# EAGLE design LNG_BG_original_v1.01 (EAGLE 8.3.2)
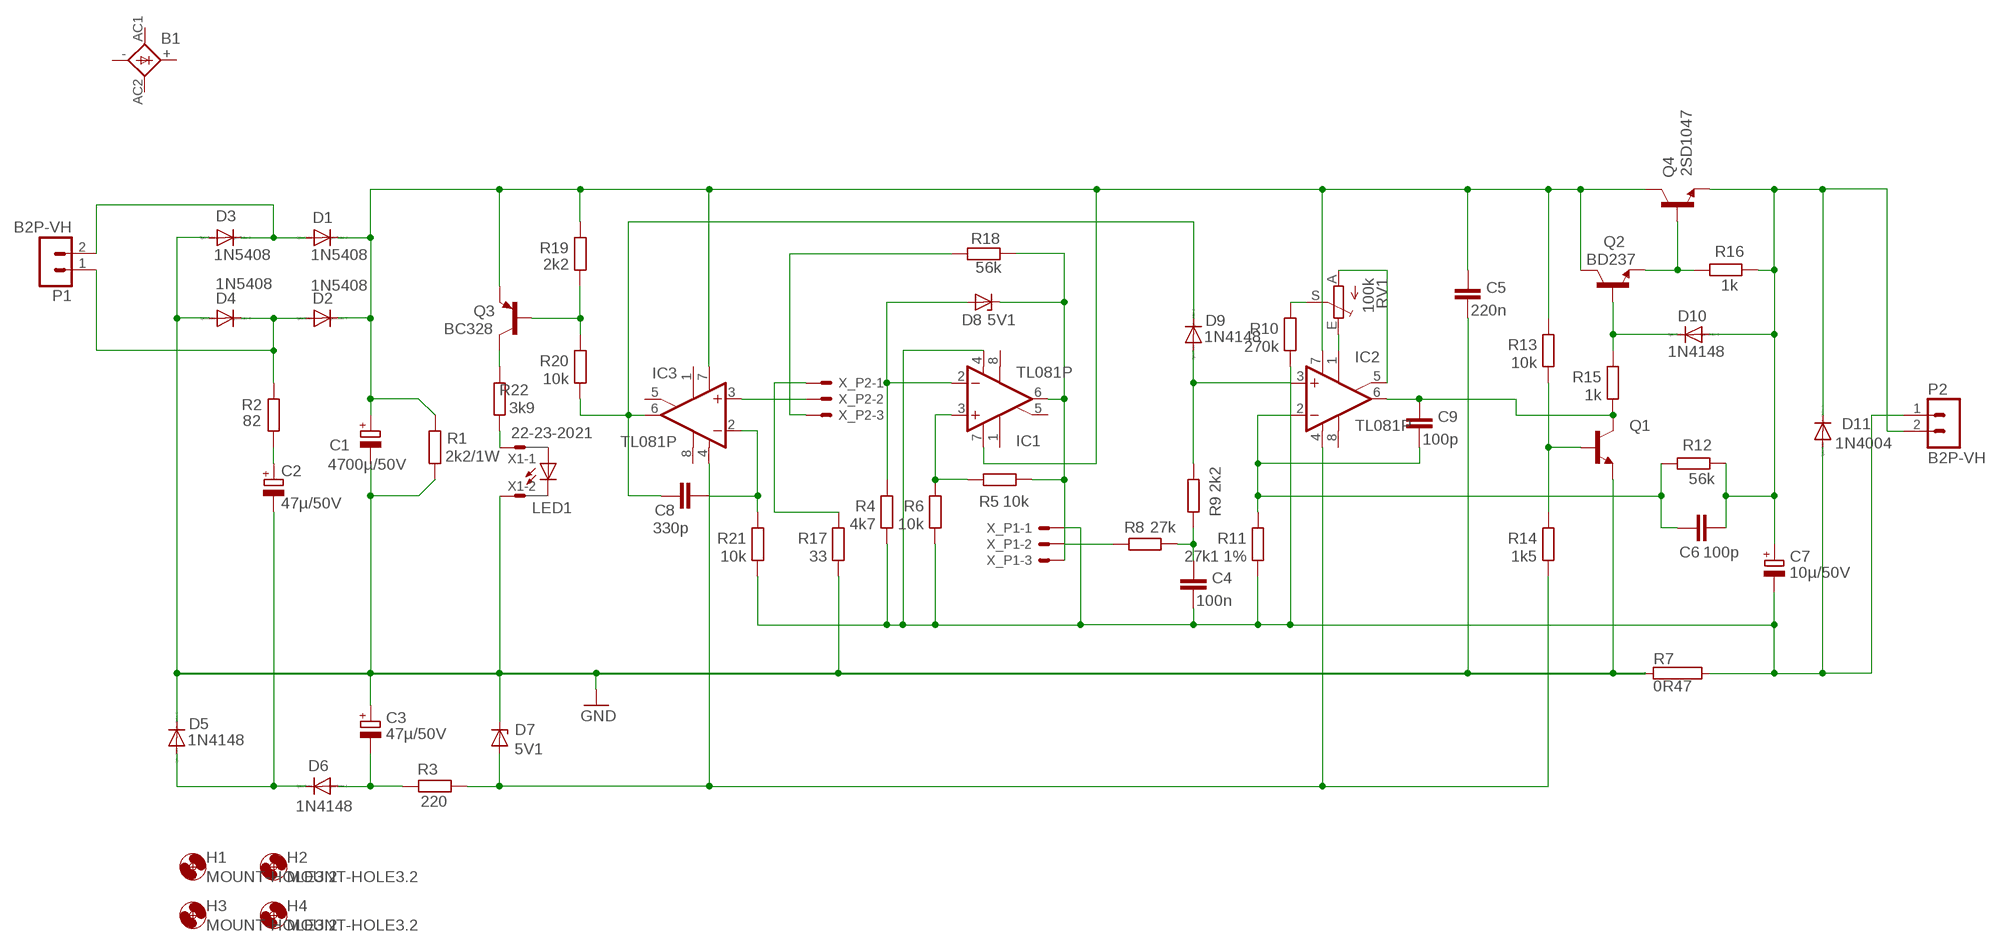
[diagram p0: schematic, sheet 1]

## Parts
B1  DSI32A  [DSI32A]
C1  4700µ/50V  CPOL-EUE7.5-18  [E7,5-18]
C2  47µ/50V  CPOL-EUE2.5-6  [E2,5-6]
C3  47µ/50V  CPOL-EUE2.5-6  [E2,5-6]
C4  100n  C-EU050-024X044  [C050-024X044]
C5  220n  C-EU050-024X044  [C050-024X044]
C6  100p  C-EU050-024X044  [C050-024X044]
C7  10µ/50V  CPOL-EUE2.5-6  [E2,5-6]
C8  330p  C-EU050-024X044  [C050-024X044]
C9  100p  C-EU050-024X044  [C050-024X044]
D1  1N5408  1N5400  [DO201-15]
D2  1N5408  1N5400  [DO201-15]
D3  1N5408  1N5400  [DO201-15]
D4  1N5408  1N5400  [DO201-15]
D5  1N4148  1N4148DO35-10  [DO35-10]
D6  1N4148  1N4148DO35-10  [DO35-10]
D7  5V1  BZV10  [DO34Z7]
D8  5V1  BZV10  [DO34Z7]
D9  1N4148  1N4148DO35-10  [DO35-10]
D10  1N4148  1N4148DO35-10  [DO35-10]
D11  1N4004  [DO41-10]
H1  MOUNT-HOLE3.2  [3,2]
H2  MOUNT-HOLE3.2  [3,2]
H3  MOUNT-HOLE3.2  [3,2]
H4  MOUNT-HOLE3.2  [3,2]
IC1  TL081P  [DIL08]
IC2  TL081P  [DIL08]
IC3  TL081P  [DIL08]
LED1  LED3MM  [LED3MM]
P1  B2P-VH  [B2P-VH]
P2  B2P-VH  [B2P-VH]
Q1  BC337-NPN-TO92-CBE  [TO92-CBE]
Q2  BD237  BD235  [TO126]
Q3  BC328  [TO92-EBC]
Q4  2SD1047  2SC3855  [SC-65]
R1  2k2/1W  R-EU_0414/15  [0414/15]
R2  82  R-EU_0207/10  [0207/10]
R3  220  R-EU_0207/10  [0207/10]
R4  4k7  R-EU_0207/10  [0207/10]
R5  10k  R-EU_0207/10  [0207/10]
R6  10k  R-EU_0207/10  [0207/10]
R7  0R47  RKH208-8  [KH208-8]
R8  27k  R-EU_0207/10  [0207/10]
R9  2k2  R-EU_0207/10  [0207/10]
R10  270k  R-EU_0207/10  [0207/10]
R11  27k1 1%  R-EU_0207/10  [0207/10]
R12  56k  R-EU_0207/10  [0207/10]
R13  10k  R-EU_0207/10  [0207/10]
R14  1k5  R-EU_0207/10  [0207/10]
R15  1k  R-EU_0207/10  [0207/10]
R16  1k  R-EU_0207/10  [0207/10]
R17  33  R-EU_0207/10  [0207/10]
R18  56k  R-EU_0207/10  [0207/10]
R19  2k2  R-EU_0207/10  [0207/10]
R20  10k  R-EU_0207/10  [0207/10]
R21  10k  R-EU_0207/10  [0207/10]
R22  3k9  R-EU_0207/10  [0207/10]
RV1  100k  TRIM_EU-B64Y  [B64Y]
X1  22-23-2021  [22-23-2021]
X_P1  22-23-2031  [22-23-2031]
X_P2  22-23-2031  [22-23-2031]

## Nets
GND: C1.- C3.+ C5.2 D3.A D4.A D5.C D7.C Q1.E R1.1 R7.1 R17.1 X1.2
N$1: D1.A D3.C P1.2
N$2: D2.A D4.C P1.1 R2.1
N$3: C2.+ R2.2
N$4: C9.1 IC2.6(OUT) Q1.C R15.1
N$5: C2.- D5.A D6.C
N$6: Q3.B R19.1 R20.2
N$7: C3.- D6.A R3.1
N$8: C1.+ C5.1 D1.C D2.C IC1.7(V+) IC2.7(V+) IC3.7(V+) Q2.2(C) Q3.E Q4.2(C) R1.2 R13.2 R19.2
N$9: C8.2 D9.C IC3.6(OUT) R20.1
N$10: C8.1 IC3.2(-IN) R21.2
N$11: R22.1 X1.1
N$12: Q3.C R22.2
N$13: D7.A IC2.4(V-) IC3.4(V-) R3.2 R14.1
N$14: IC3.3(+IN) X_P2.2
N$15: R17.2 X_P2.1
N$16: R18.2 X_P2.3
N$17: IC1.3(+IN) R5.2 R6.2
N$18: R8.2 X_P1.2
N$19: D8.A IC1.2(-IN) R4.2
N$20: D8.C IC1.6(OUT) R5.1 R18.1 X_P1.3
N$21: C4.1 R8.1 R9.2
N$22: D9.A IC2.3(+IN) R9.1
N$23: C6.2 C7.+ D10.A D11.C P2.2 Q4.3(E) R12.1 R16.1
N$24: R10.2 RV1.S
N$25: IC2.1(ON1) RV1.E
N$26: IC2.5(ON2) RV1.A
N$28: Q1.B R13.1 R14.2
N$29: D10.C Q2.3(B) R15.2
N$31: Q2.1(E) Q4.1(B) R16.2
N$32: C4.2 C7.- D11.A IC1.4(V-) P2.1 R4.1 R6.1 R7.2 R10.1 R11.1 R21.1 X_P1.1
N$35: C6.1 C9.2 IC2.2(-IN) R11.2 R12.2
Unconnected: B1.+ B1.- B1.AC1 B1.AC2 IC1.1(ON1) IC1.5(ON2) IC1.8(OPT) IC2.8(OPT) IC3.1(ON1) IC3.5(ON2) IC3.8(OPT) LED1.A LED1.K(C)

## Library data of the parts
B1 = rectifier:DSI32A: RECTIFIER 3.2 A
C1-C3 C7 = rcl:CPOL-EU: POLARIZED CAPACITOR, European symbol
C4-C6 C8 C9 = rcl:C-EU: CAPACITOR, European symbol
D1-D4 = diode:1N5400: DIODE
D5 D6 D9 D10 = diode:1N4148: DIODE
D7 D8 = diode:BZV10: Z DIODE
D11 = diode:1N4004: DIODE
H1-H4 = holes:MOUNT-HOLE: MOUNTING HOLE with drill center marker
IC1-IC3 = linear:TL081: OP AMP
LED1 = led:LED: LED
P1 P2 = con-jst-vh:B2P-VH: HEADER
Q1 = transistor:*-NPN-: NPN Transistror BF959 corrected 2008.03.06
Q2 = transistor:BD235: NPN TRANSISTOR
Q3 = transistor-pnp:BC328*: PNP Transistror
Q4 = transistor-JP:2SC3855: NPN Power Transistor 140V, 10A, 100W
R1-R6 R8-R22 = rcl:R-EU_: RESISTOR, European symbol
R7 = resistor-power:R: Power Resitor; OC_FARNELL: unknown; OC_NEWARK: unknown
RV1 = pot:TRIM_EU-: POTENTIOMETER
X1 = con-molex:22-23-2021: .100" (2.54mm) Center Header - 2 Pin; MF: MOLEX; MPN: 22-23-2021; OC_FARNELL: 1462926; OC_NEWARK: 25C3832
X_P1 X_P2 = con-molex:22-23-2031: .100" (2.54mm) Center Header - 3 Pin; MF: MOLEX; MPN: 22-23-2031; OC_FARNELL: 1462950; OC_NEWARK: 30C0862

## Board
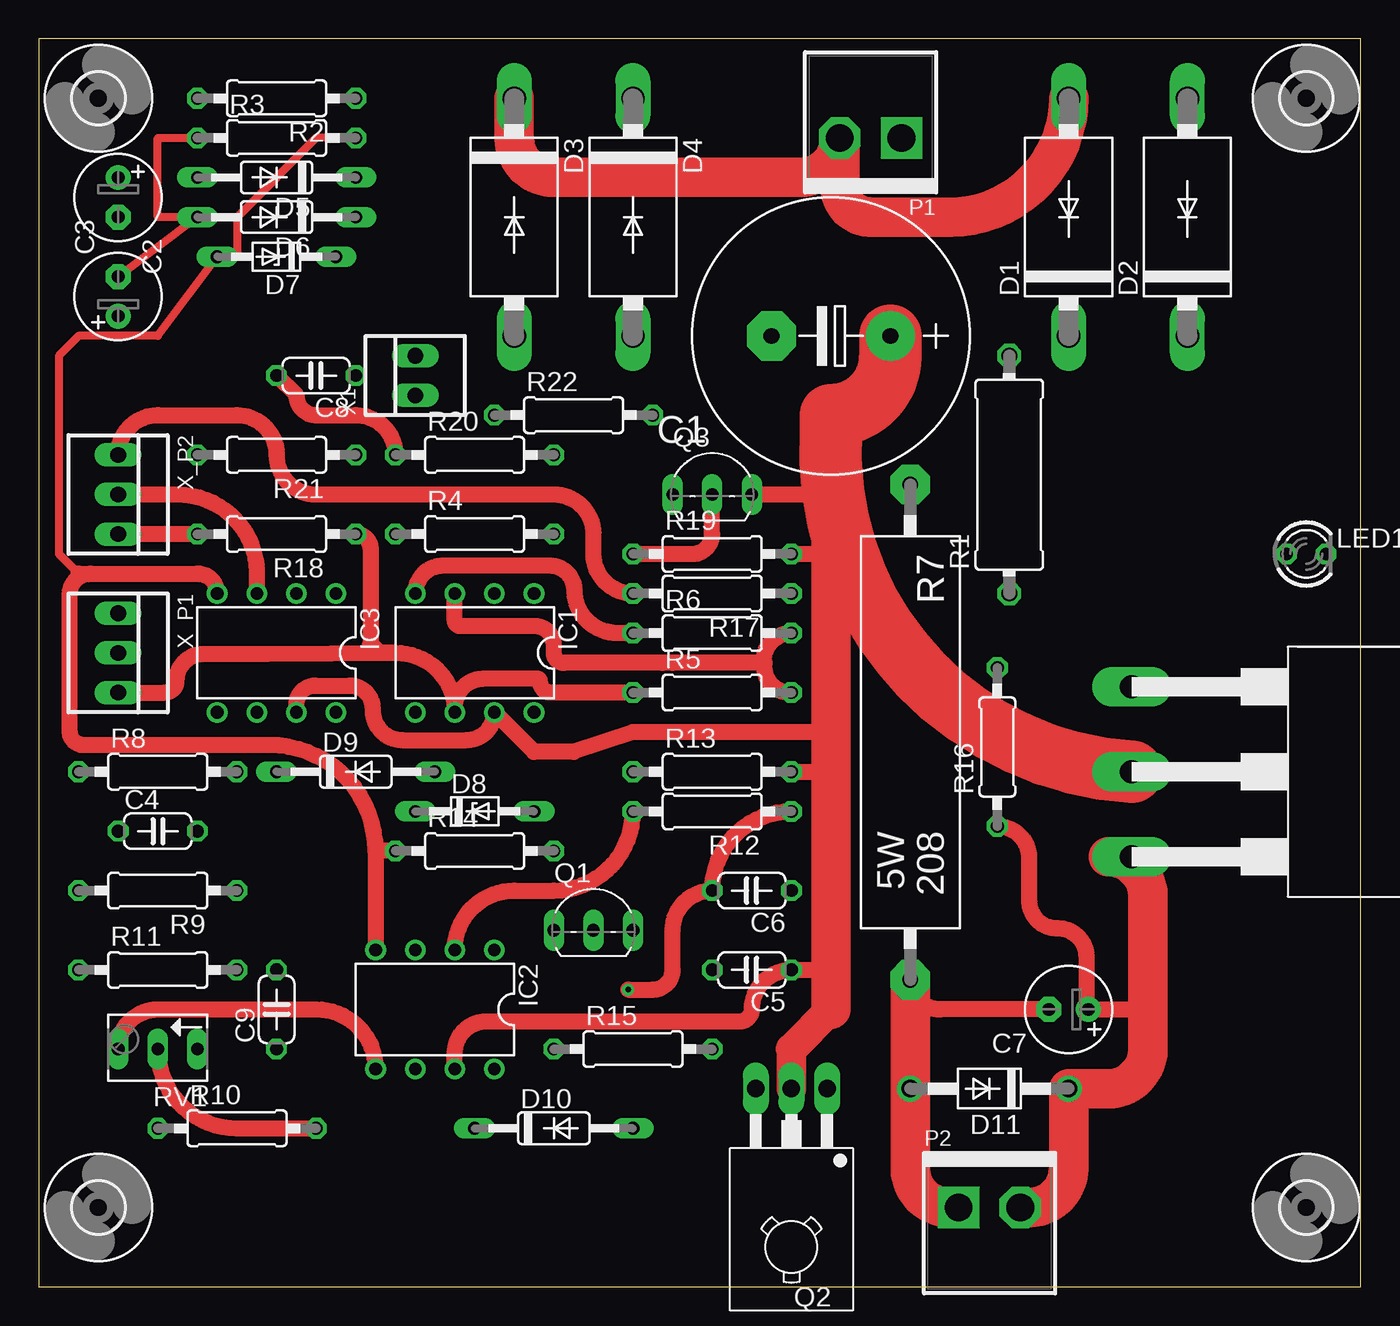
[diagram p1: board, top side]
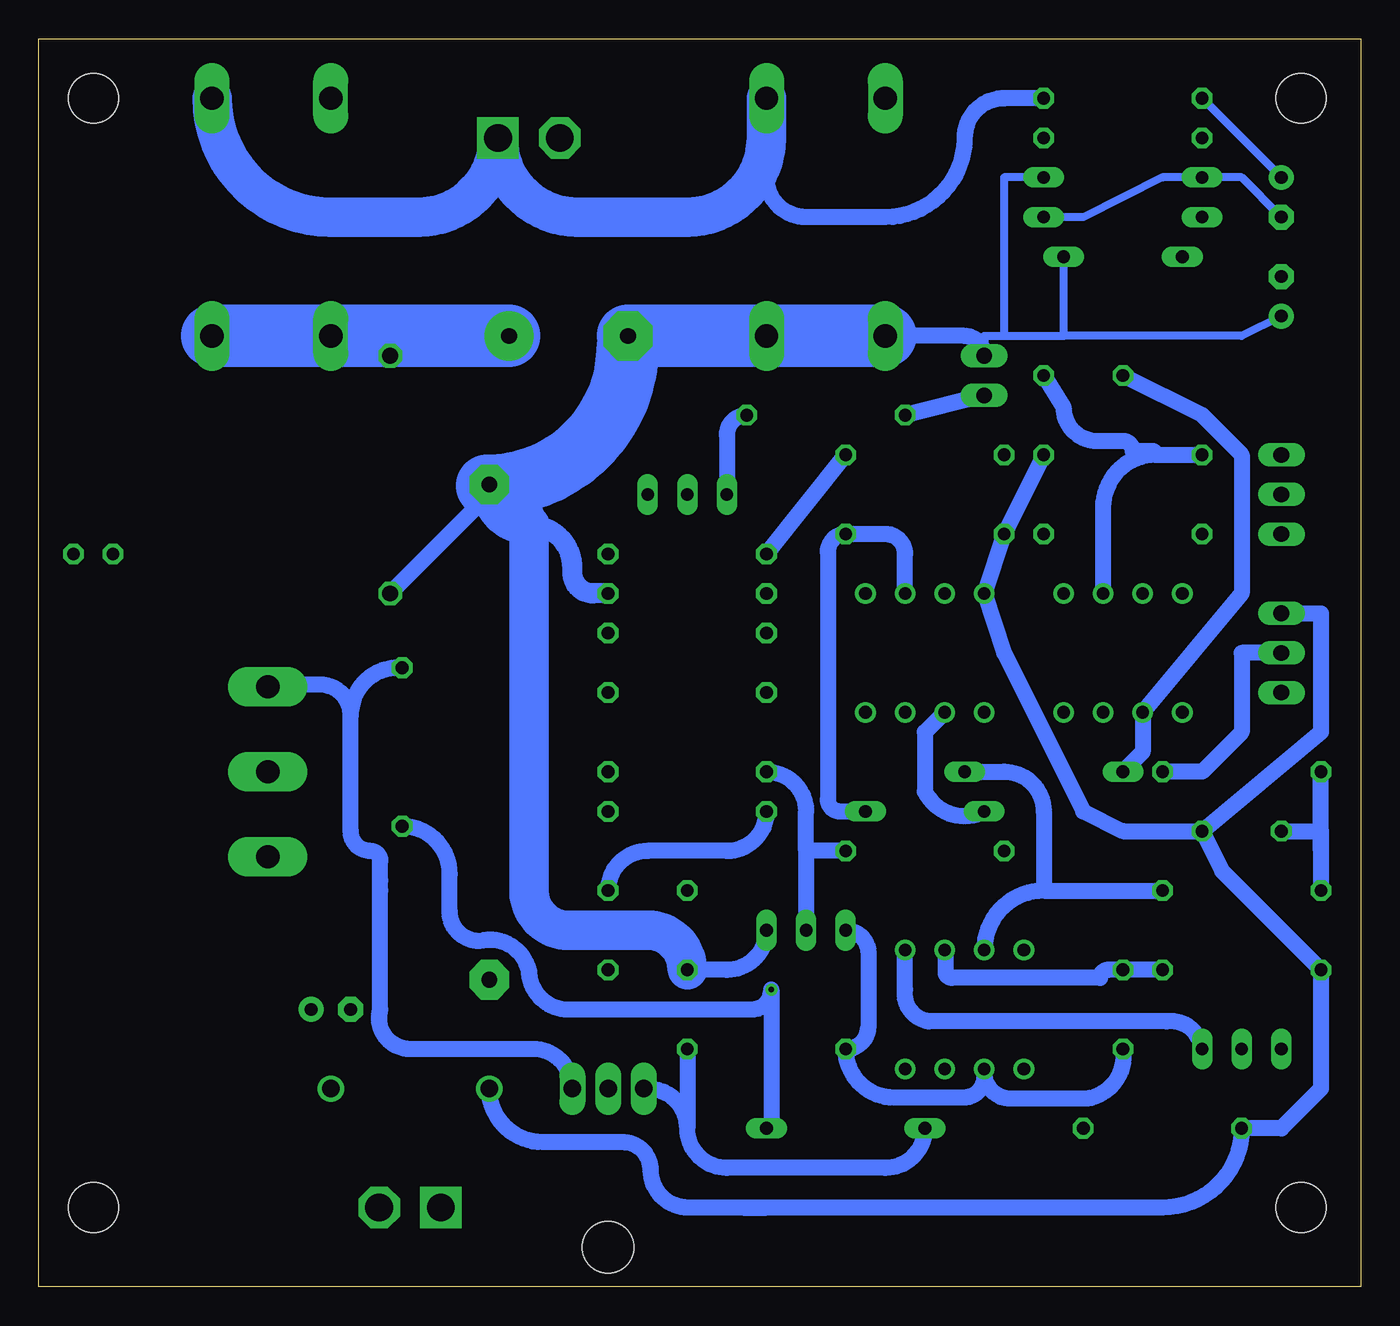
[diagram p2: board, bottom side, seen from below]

Size 84.76 x 80 mm. Coordinates in mm from the lower left corner, seen from the top.
Outline: 0,0 84.76,0 84.76,80 0,80 0,0
Copper layers (1*16): Top 0.035mm / dielectric 1.5mm / Bottom 0.035mm
Design rules "default": minimum track width 6mil, minimum drill 0.35mm, track to track 6mil, track to pad 6mil, pad to pad 6mil, via to via 6mil, smd to smd 6mil, copper to edge 40mil, drill to drill 6mil, minimum pad ring 10mil, minimum via ring 8mil, stop-mask expansion 4mil, vias tented up to drill 0mil, thermal gap 10mil

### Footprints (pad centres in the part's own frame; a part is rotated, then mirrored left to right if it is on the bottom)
DSI32A = drill 1.321 long: + -3.982,1.5; - 11.004,1.5; AC1 -11.5,1.5; AC2 3.511,1.5
E7,5-18 = drill 1.016 pad 3.15: + -3.81,0 | drill 1.016 pad 3.15 octagon: - 3.81,0
E2,5-6 = drill 0.813 pad 1.6: + -1.27,0 | drill 0.813 pad 1.6 octagon: - 1.27,0
C050-024X044 = drill 0.813 octagon: 1 -2.54,0; 2 2.54,0
DO201-15 = drill 1.499 long: A 7.62,0; C -7.62,0
DO35-10 = drill 0.813 long: A 5.08,0; C -5.08,0
DO34Z7 = drill 0.813 long: A 3.81,0; C -3.81,0
DO41-10 = drill 1.118: A 5.08,0; C -5.08,0
3,2 = hole 3.2: 0,0
DIL08 = drill 0.813 pad 1.27: 1 -3.81,-3.81; 2 -1.27,-3.81; 3 1.27,-3.81; 4 3.81,-3.81; 5 3.81,3.81; 6 1.27,3.81; 7 -1.27,3.81; 8 -3.81,3.81
LED3MM = drill 0.813 octagon: A -1.27,0; K 1.27,0
B2P-VH = drill 1.778 square: 1 -1.98,0 | drill 1.778 octagon: 2 1.98,0
TO92-CBE = drill 0.813 long: B 0,0; C -2.54,0; E 2.54,0
TO126 = drill 1.118 long: 1 -2.286,-5.08; 2 0,-5.08; 3 2.286,-5.08 | hole 3.302: 0,5.08
TO92-EBC = drill 0.813 long: B 0,-1.27; C -2.54,-1.27; E 2.54,-1.27
SC-65 = drill 1.5 pad 2.54 long: 1 -5.45,-18.81; 2 0,-18.81; 3 5.45,-18.81
0414/15 = drill 1.016 octagon: 1 -7.62,0; 2 7.62,0
0207/10 = drill 0.813 octagon: 1 -5.08,0; 2 5.08,0
KH208-8 = drill 1.016 pad 2.54 octagon: 1 -15.875,0; 2 15.875,0
B64Y = drill 0.813 long: A 2.54,0; E -2.54,0; S 0,0
22-23-2021 = drill 1 long: 1 -1.27,0; 2 1.27,0
22-23-2031 = drill 1 long: 1 -2.54,0; 2 0,0; 3 2.54,0

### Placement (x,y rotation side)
B1  not placed on the board
C1  50.8,60.96 180 top
C2  5.08,69.85 270 top
C3  5.08,63.5 90 top
C4  7.62,29.21 0 top
C5  45.72,20.32 180 top
C6  45.72,25.4 180 top
C7  66.04,17.78 180 top
C8  17.78,58.42 180 top
C9  15.24,17.78 90 top
D1  66.04,68.58 90 top
D2  73.66,68.58 90 top
D3  30.48,68.58 270 top
D4  38.1,68.58 270 top
D5  15.24,71.12 180 top
D6  15.24,68.58 180 top
D7  15.24,66.04 180 top
D8  27.94,30.48 0 top
D9  20.32,33.02 0 top
D10  33.02,10.16 0 top
D11  60.96,12.7 180 top
H1  3.81,76.2 0 top
H2  3.81,5.08 0 top
H3  81.28,5.08 0 top
H4  81.28,76.2 0 top
IC1  27.94,40.64 180 top
IC2  25.4,17.78 180 top
IC3  15.24,40.64 180 top
LED1  81.28,46.99 0 top
P1  53.34,73.66 180 top
P2  60.96,5.08 0 top
Q1  35.56,22.86 0 top
Q2  48.26,7.62 180 top
Q3  43.18,52.07 0 top
Q4  88.9,33.02 270 top
R1  62.23,52.07 90 top
R2  15.24,76.2 180 top
R3  15.24,73.66 0 top
R4  27.94,48.26 0 top
R5  43.18,38.1 0 top
R6  43.18,41.91 0 top
R7  55.88,35.56 270 top
R8  7.62,33.02 0 top
R9  7.62,25.4 180 top
R10  12.7,10.16 0 top
R11  7.62,20.32 0 top
R12  43.18,30.48 180 top
R13  43.18,33.02 0 top
R14  27.94,27.94 0 top
R15  38.1,15.24 0 top
R16  61.47,34.61 90 top
R17  43.18,44.45 180 top
R18  15.24,48.26 180 top
R19  43.18,46.99 0 top
R20  27.94,53.34 0 top
R21  15.24,53.34 180 top
R22  34.29,55.88 0 top
RV1  7.62,15.24 180 top
X1  24.13,58.42 90 top
X_P1  5.08,40.64 270 top
X_P2  5.08,50.8 270 top

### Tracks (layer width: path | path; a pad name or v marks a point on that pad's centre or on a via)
GND
  Bottom 0.508: C3.+ 7.62,60.96 19.05,60.96 | 22.86,60.96 19.05,60.96 | 22.86,60.96 24.13,60.96 X1.2 | D7.C 19.05,60.96 | D5.C 22.86,71.12 22.86,60.96
  Bottom 1.016: R1.1 55.88,50.8 R7.1 arc-90 55.37,50.93 | Q1.E arc90 40.64,20.32 C5.2 | X1.2 arc-90 25.4,60.96 D3.A
  Bottom 1.27: R17.1 49.21,44.45 arc90 50.55,45.78 50.55,46.1 arc-90 53.28,48.83
  Bottom 2.54: C1.- 46.99,60.33 | 56.01,51.37 R7.1 arc-90 53.28,48.83 | C5.2 arc-90 45.72,22.86 50.8,22.86 arc90 53.34,25.4 53.34,48.26 arc-90 55.88,50.8
  Bottom 4: D3.A D4.A C1.- | 56.01,51.37 arc-90 46.99,60.33
N$1
  Top 2.54: D3.C 30.48,73.66 arc90 33.02,71.12 48.82,71.12 arc90 P1.2 51.36,70.56 arc90 53.34,68.58 58.42,68.58 arc90 D1.A
N$2
  Bottom 1.016: R2.1 22.86,76.2 arc-90 25.4,73.66 arc90 30.48,68.58 35.56,68.58 arc90 38.1,71.12 38.1,73.66
  Bottom 2.54: D2.A arc-90 66.04,68.58 60.4,68.58 arc-90 P1.1 arc-90 50.24,68.58 43.18,68.58 arc-90 38.1,73.66 D4.C
N$3
  Bottom 0.508: R2.2 C2.+
N$4
  Bottom 1.016: C9.1 arc90 17.53,12.06 22.61,12.06 arc90 IC2.6 24.13,13.46 arc90 25.46,12.13 29.91,12.13 arc90 R15.1 arc-90 31.56,16.7 31.56,21.4 arc-90 Q1.C
N$5
  Bottom 0.508: C2.- 7.62,71.12 D5.A 12.7,71.12 17.78,68.58 D6.C
N$6
  Top 1.016: R19.1 41.91,46.99 arc90 43.18,48.26 Q3.B
  Bottom 1.016: R20.2 R19.1
N$7
  Top 0.508: C3.- D6.A 7.62,68.58 7.62,73.66 R3.1
N$8
  Top 1.016: R19.2 50.8,46.99 | R13.2 50.8,33.02 | 50.8,35.56 38.1,35.56 34.29,34.29 31.75,34.29 IC1.7 arc-90 27.43,35.05 23.3,35.05 arc-90 21.4,36.96 21.4,37.08 arc90 19.94,38.54 17.72,38.54 arc90 16.51,37.34 IC3.7 | IC2.7 26.67,14.99 arc-90 28.7,17.02 44.96,17.02 arc90 45.72,17.78 arc-90 C5.1 50.8,20.32 | Q3.E 50.8,50.8
  Top 1.9: Q2.2 48.26,15.24
  Top 2: 50.8,17.78 48.26,15.24
  Top 2.54: 50.8,54.85 50.8,50.8 50.8,46.99 50.8,35.56 50.8,33.02 50.8,20.32 50.8,17.78
  Top 4: Q4.2 arc-90 50.8,54.85 50.8,55.88 arc90 54.61,59.69 C1.+
  Bottom 1.016: R1.2 arc-90 63.5,60.96
  Bottom 4: D2.C D1.C 63.5,60.96 C1.+
N$9
  Top 1.016: C8.2 16.51,57.15 arc90 17.78,55.88 20.32,55.88 arc-90 R20.1
  Bottom 1.016: D9.C 13.97,34.29 IC3.6 7.62,44.45 7.62,53.34 10.16,55.88 C8.2
N$10
  Bottom 1.016: 13.14,53.34 R21.2 | 13.14,53.34 arc-90 16.51,49.97 IC3.2 | C8.1 19.05,56.39 arc-90 16.89,54.23 15.24,54.23 arc90 14.61,53.59 13.4,53.59 arc90 13.14,53.34
N$11
  Bottom 1.016: X1.1 R22.1
N$12
  Bottom 1.016: R22.2 arc-90 40.64,54.61 Q3.C
N$13
  Top 0.508: R3.2 17.78,73.66 12.7,68.58 12.7,66.04 D7.A 7.62,60.96 2.54,60.96 1.27,59.69 1.27,46.99 2.54,45.72 3.3,45.72
  Top 1.016: 21.59,27.94 IC2.4 | 21.59,27.94 arc90 14.8,34.73 2.86,34.73 arc-90 1.97,35.62 1.97,44.39 arc-90 3.3,45.72 | 2.54,45.72 10.16,45.72 arc-90 IC3.4 | R14.1 21.59,27.94
N$14
  Top 1.016: X_P2.2 8.89,50.8 arc-90 13.97,45.72 IC3.3
N$15
  Top 1.016: R17.2 arc-90 35.56,46.99 35.56,48.26 arc90 33.02,50.8 17.78,50.8 arc-90 15.24,53.34 arc90 12.7,55.88 7.62,55.88 arc90 X_P2.1
N$16
  Top 1.016: R18.2 X_P2.3
N$17
  Top 1.016: IC1.3 26.67,42.74 arc90 27.05,42.35 31.81,42.35 arc-90 33.02,41.15 33.02,40.64 arc90 33.66,40.01 40.64,40.01 | R5.2 47.94,38.1 arc-90 46.55,40.01 | 46.55,40.01 46.48,40.13 arc-90 R6.2 | 46.55,40.01 40.64,40.01 | 40.64,40.01 40.01,40.01
N$18
  Bottom 1.016: X_P1.2 7.62,40.64 7.62,35.56 10.16,33.02 R8.2
N$19
  Bottom 1.016: D8.A 33.4,30.48 arc90 34.16,31.24 34.16,47.12 arc90 R4.2 30.48,48.26 arc90 29.21,46.99 IC1.2
N$20
  Top 1.016: R5.1 32.83,38.1 arc-90 32.13,38.8 arc90 31.94,38.99 28.51,38.99 arc90 26.67,37.15 | 26.67,37.15 IC1.6 | X_P1.3 8.06,38.1 arc90 8.83,38.86 arc-90 10.54,40.58 arc1 22.86,40.64 | 22.86,40.64 arc-86 26.67,37.15 | R18.1 arc-90 21.27,47.31 21.27,41.21 | 21.27,41.21 21.21,41.15 | 22.86,40.64 21.84,40.64 21.27,41.21
  Bottom 1.016: IC1.6 27.94,35.56 27.94,31.75 arc-90 D8.C
N$21
  Bottom 1.016: 2.54,27.94 R8.1 | 2.54,27.94 R9.2 | C4.1 2.54,29.21 2.54,27.94
N$22
  Bottom 1.016: 20.32,25.4 arc-90 IC2.3 | 20.32,25.4 R9.1 | D9.A 22.86,33.02 arc90 20.32,30.48 20.32,25.4
N$23  (via drill 0.35)
  Top 1.016: v37.78,19.05 39.37,19.05 arc90 40.64,20.32 40.64,22.86 arc-90 C6.2 arc-90 R12.1 | R16.1 arc-90 63.5,27.5 63.5,24.77 arc90 65.28,22.99 65.34,22.99 arc-90 67.18,21.14 67.18,17.91 arc90 C7.+ 71.12,17.78
  Top 2.54: P2.2 63.5,5.08 arc90 66.04,7.62 D11.C 68.58,12.7 arc90 71.12,15.24 71.12,17.78 71.12,25.03 arc90 68.58,27.57 Q4.3
  Bottom 1.016: D10.A arc-90 37.78,10.48 v37.78,19.05 arc90 39.05,17.78 50.8,17.78 arc90 53.34,20.32 arc-90 56.52,22.16 arc90 58.42,24.07 58.42,26.48 arc-90 R16.1
N$24
  Top 1.016: RV1.S arc90 12.7,10.16 R10.2
N$25
  Bottom 1.016: RV1.E arc-90 12.45,17.02 27.69,17.02 arc90 29.21,19.05 IC2.1
N$26
  Top 1.016: RV1.A arc-90 7.62,17.78 17.78,17.78 arc-90 IC2.5
N$28
  Bottom 1.016: R13.1 arc90 35.56,30.48 35.56,27.94 | 35.56,27.94 Q1.B | R14.2 35.56,27.94
N$29
  Bottom 1.016: Q2.3 45.72,12.7 arc90 43.18,10.16 | R15.2 43.18,10.16 | D10.C arc90 30.48,7.62 40.64,7.62 arc90 43.18,10.16
N$31
  Bottom 1.016: 62.87,25.4 62.87,17.78 arc-106 60.96,15.24 53.09,15.24 arc90 Q2.1 | 62.87,25.4 62.87,26.04 | 62.87,25.4 62.87,27.3 arc-90 63.5,27.94 arc90 64.77,29.21 64.77,36.64 | 64.77,36.64 arc-90 66.74,38.61 69.95,38.61 arc-90 Q4.1 | R16.2 61.72,39.69 arc-90 64.77,36.64
N$32
  Top 1.016: R6.1 37.08,41.91 arc-90 34.35,44.64 arc90 32.77,46.23 25.91,46.23 arc90 IC1.4 | C7.- 57.78,17.78 arc-90 R7.2
  Top 2.54: P2.1 58.42,5.08 arc-90 55.88,7.62 D11.A R7.2
  Bottom 1.016: X_P1.1 2.54,43.18 2.54,35.56 C4.2 | C4.2 8.89,26.67 R11.1 2.54,12.7 5.08,10.16 R10.1 arc90 12.7,5.08 38.1,5.08 | C4.2 15.24,29.21 17.78,30.48 22.86,40.64 IC1.4 R4.1 R21.1 | 39.61,5.08 38.1,5.08 | 39.61,5.08 43.12,5.08 arc90 45.53,7.49 arc-90 47.31,9.27 48.26,9.27 | 48.26,9.27 48.32,9.27 | 48.26,9.27 52.45,9.27 arc90 D11.A | 38.1,5.08 39.61,5.08
N$35
  Top 1.016: IC2.2 arc-90 30.48,25.4 33.02,25.4 arc90 R12.2
  Bottom 1.016: R11.2 C9.2 16.19,20.32 arc-90 16.7,19.81 26.23,19.81 arc90 26.61,20.19 26.61,21.53 arc-90 IC2.2 | R12.2 arc90 40.64,27.94 45.72,27.94 arc-90 C6.1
